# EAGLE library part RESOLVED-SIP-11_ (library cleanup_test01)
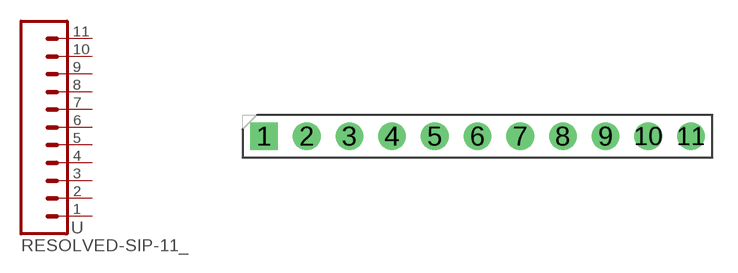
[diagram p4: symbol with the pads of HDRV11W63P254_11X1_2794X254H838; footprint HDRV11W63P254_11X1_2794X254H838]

Designator prefix -

## RESOLVED-SIP-11_2.54-SPACE-VERTICAL  [HDRV11W63P254_11X1_2794X254H838]
1  1  pas
2  2  pas
3  3  pas
4  4  pas
5  5  pas
6  6  pas
7  7  pas
8  8  pas
9  9  pas
10  10  pas
11  11  pas

## Footprint HDRV11W63P254_11X1_2794X254H838 (pad centres in mm)
drill 1.1 pad 1.65 square: 1 0,0
drill 1.1 pad 1.65: 2 2.54,0; 3 5.08,0; 4 7.62,0; 5 10.16,0; 6 12.7,0; 7 15.24,0; 8 17.78,0; 9 20.32,0; 10 22.86,0; 11 25.4,0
